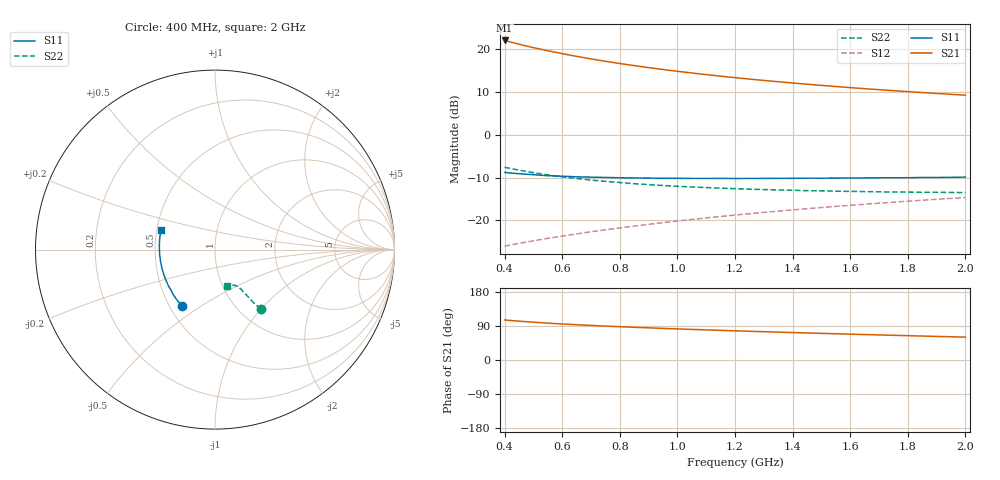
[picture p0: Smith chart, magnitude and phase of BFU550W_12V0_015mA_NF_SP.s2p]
! Filename:  P:\Prog\Test\Noise\ATS_data\Testdata_Net\06 Compressed Noise after Statistics\BFU550W_APM2013_11_D05_12p0V_015mA_NF_CM01_D.sf
! Date/Time: Tue 26/Mar/2013 16:25:21
! BFU550W_APM2013_11_D05_12p0V_1to35mA_NF_CM01_Bias7_R.sf
! Noise Parameter Data File
! BFU550W_APM2013_11_D05_12p0V_1to35mA_NF_CM01
! Date/time: Mon Mar 25 15:58:35 2013
! VAR V_out= 12.001000
! VAR I_out= 14.990000
! VAR V_in= 0.782200
! VAR I_in= 0.133800
! Device data file deembeded for feedlines and parallel
! Original file: \06 Compressed Noise after Statistics\BFU550W_APM2013_11_D05_12p0V_015mA_NF_CM01_R.sf
! Feed-files: PR019V01_070313_Feed1.s2p, PR019V01_070313_Feed2.s2p
! Parallel-file: PR019V01_070313_Par.s2p
# MHz S MA R 50
!  Freq-MHz  S11-mag  S11-arg  S21-mag  S21-arg  S12-mag  S12-arg  S22-mag  S22-arg
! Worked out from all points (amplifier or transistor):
!   37 points, 400 MHz to 2 GHz, reference 50 ohm
!   highest |S21| = 22.1 dB at 400 MHz (marker M1)
!   |S21| within 3 dB of that: start of sweep to 594.1 MHz
!   unconditionally stable (mu >= 1): 1.299 GHz to end of sweep
!   at 500 MHz: K = 0.82, MSG = 22.6 dB, |S12| = -24.8 dB
!   at 1.1 GHz: K = 0.99, MSG = 16.8 dB, |S12| = -19.4 dB
!   at 2 GHz: K = 1.01, MAG = 11.4 dB, |S12| = -14.6 dB
!   lowest NFmin = 0.84 dB at 420 MHz
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400  0.3635 -120.4  12.69 105.7  0.04999 61.7  0.4177 -52.4
420  0.3584 -123.2  12.17 104.3  0.05156 61.9  0.4051 -52.8
433  0.355 -124.8  11.86 103.5  0.05255 62.0  0.397 -53.1
460  0.3495 -128.2  11.25 102.0  0.05463 62.4  0.3817 -53.5
500  0.3422 -132.9  10.46 99.8  0.05773 62.8  0.3617 -54.1
550  0.333 -137.8  9.626 97.3  0.06164 63.4  0.3405 -54.5
600  0.3285 -142.5  8.899 95.1  0.0656 63.9  0.3227 -54.9
650  0.3232 -146.5  8.269 93.1  0.06958 64.4  0.3088 -55.3
700  0.3203 -150.3  7.723 91.2  0.07364 64.8  0.2963 -55.6
750  0.3177 -153.7  7.245 89.5  0.07769 65.2  0.2857 -55.9
800  0.3152 -157.0  6.822 87.8  0.0818 65.5  0.2771 -56.4
850  0.3137 -160.1  6.446 86.3  0.08588 65.8  0.2685 -56.5
950  0.3106 -165.2  5.808 83.4  0.09423 66.2  0.2559 -57.2
1050  0.3097 -169.9  5.287 80.7  0.1027 66.5  0.246 -58.1
1150  0.31 -174.3  4.853 78.2  0.1111 66.5  0.2382 -59.0
1200  0.3092 -176.1  4.666 77.0  0.1155 66.5  0.2351 -59.6
1250  0.3095 -178.2  4.488 75.8  0.1197 66.5  0.2318 -60.0
1350  0.3101 178.5  4.178 73.6  0.1284 66.3  0.2267 -61.2
1500  0.3114 173.4  3.787 70.3  0.1414 65.9  0.2216 -63.4
1650  0.3136 168.9  3.467 67.2  0.1545 65.4  0.2172 -65.5
1750  0.3156 166.3  3.287 65.2  0.1633 65.0  0.2147 -67.2
2000  0.3207 159.8  2.91 60.3  0.1852 63.7  0.2115 -71.9
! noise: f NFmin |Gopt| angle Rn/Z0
400  0.8893  0.1569  176  0.0802
460  0.8855  0.1677  178.5  0.0794
600  0.924  0.1709  177.2  0.0809
800  0.9408  0.1952  -179.1  0.0764
1000  0.9751  0.2091  -177.1  0.0754
1200  1.019  0.2293  -173.1  0.0744
1400  1.022  0.2503  -170.6  0.0745
1600  1.051  0.272  -170.3  0.0703
1800  1.079  0.2882  -166.4  0.0721
2000  1.099  0.3131  -157.4  0.0748
